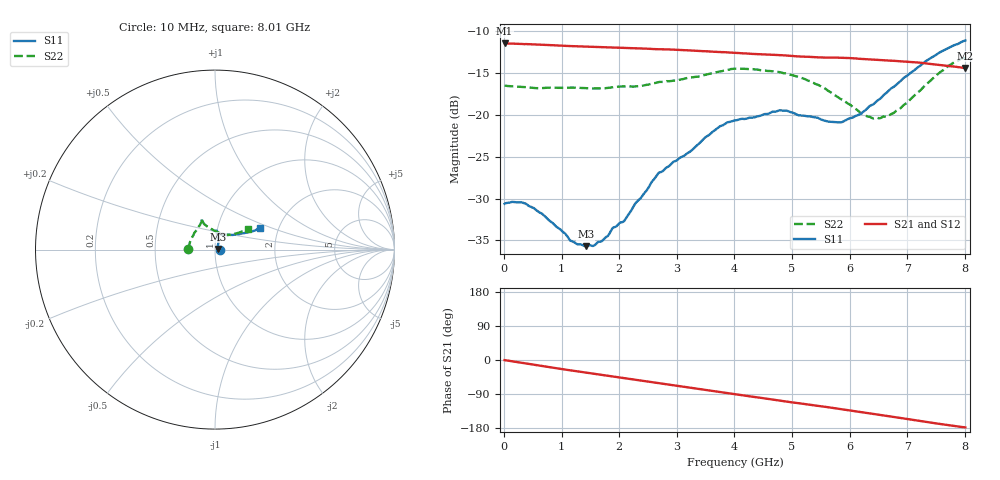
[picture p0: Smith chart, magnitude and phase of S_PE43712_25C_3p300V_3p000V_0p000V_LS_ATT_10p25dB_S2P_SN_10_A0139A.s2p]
! DEVICE ID: PE43712
! File Path: z:\PE43713\PE43713_CHAR_NOM_04292014\AMB\3p300\LS_ATT_10p25dB\PE43713_AMB_3p300V_3p000V_0p000V_LS_ATT_10p25dB_S2P_SN_10_A0139A.s2p
! Serial: 10
! Lot: A0139A
! Temp: 25C
! VDD: 3.300
! VSS: 0.000
! Control_Hi: 3.000
! Control_Lo: 0.000
! Attenuation Step: 10.25dB
! Port 1: RF1
! Port 2: RF2
! ThroughPath:1-2
! IDD: 0.0001467664
! ISS: -1.594e-007
#  Hz  S  RI  R  50
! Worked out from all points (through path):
!   801 points, 10 MHz to 8.01 GHz, reference 50 ohm
!   highest |S21| = -11.43 dB at 10 MHz (marker M1); lowest = -14.4 dB at 8.01 GHz (marker M2)
!   group delay of S21, straight-line fit = 61.1 ps
!   lowest |S11| = -35.7 dB at 1.42 GHz (marker M3), VSWR 1.03, Z = 51.6 + j0.379 ohm
!   |S11| at or under -10 dB: start of sweep to end of sweep
!   |S22| runs from -20.4 to -13.1 dB; largest |S21 - S12| = 0.00099
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1e7  0.0294 0.000157  0.2683 -0.00148  0.2685 -0.00137  -0.1503 0.000982
3.7e8  0.0294 -0.00343  0.2626 -0.0421  0.2634 -0.0424  -0.1459 0.0178
6.8e8  0.025 -0.00384  0.2523 -0.075  0.2524 -0.075  -0.1413 0.033
1.17e9  0.0176 0.000478  0.2291 -0.1199  0.2291 -0.1201  -0.1352 0.0549
1.35e9  0.0165 0.00263  0.2192 -0.135  0.2192 -0.135  -0.1314 0.0619
1.42e9  0.016 0.00367  0.215 -0.1406  0.215 -0.1406  -0.1293 0.0653
1.7e9  0.0148 0.00959  0.1972 -0.1617  0.1972 -0.1617  -0.1217 0.0782
2.09e9  0.0143 0.0185  0.169 -0.1877  0.169 -0.1876  -0.1131 0.0961
2.68e9  0.0197 0.0403  0.1201 -0.2167  0.12 -0.2167  -0.0904 0.1292
3.24e9  0.0163 0.0586  0.069 -0.2334  0.069 -0.2334  -0.0791 0.1475
3.72e9  0.0145 0.083  0.0248 -0.2373  0.0247 -0.2372  -0.0745 0.1655
4.01e9  0.0115 0.0922  -0.00158 -0.2358  -0.0016 -0.2358  -0.0769 0.173
4.79e9  0.00682 0.1067  -0.0673 -0.2182  -0.0673 -0.2184  -0.0726 0.1651
5.35e9  0.0171 0.096  -0.1078 -0.1948  -0.1077 -0.1947  -0.0626 0.1445
5.88e9  0.0393 0.0822  -0.1427 -0.1676  -0.1423 -0.1677  -0.0282 0.12
6.18e9  0.0608 0.0807  -0.1592 -0.1475  -0.1589 -0.1475  -0.000754 0.1034
6.39e9  0.0805 0.0822  -0.1687 -0.133  -0.1684 -0.1329  0.0201 0.0938
6.68e9  0.1125 0.0837  -0.1803 -0.1113  -0.18 -0.1113  0.0525 0.0843
6.99e9  0.1462 0.0894  -0.19 -0.0868  -0.1897 -0.0868  0.0837 0.0832
7.36e9  0.1902 0.0987  -0.1952 -0.0557  -0.195 -0.0557  0.1254 0.0924
7.72e9  0.228 0.1093  -0.1946 -0.0272  -0.1945 -0.0274  0.1656 0.1073
8.01e9  0.252 0.121  -0.1911 -0.00705  -0.1907 -0.0074  0.1862 0.1175
